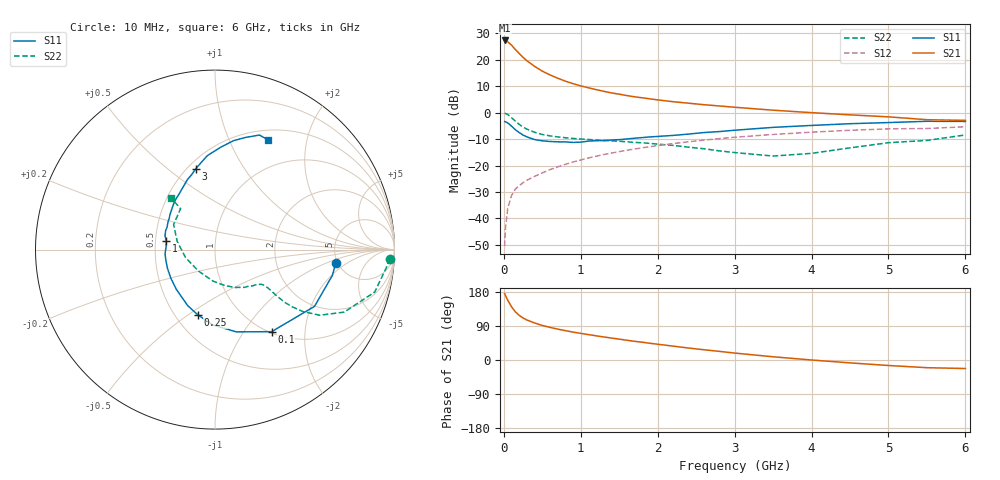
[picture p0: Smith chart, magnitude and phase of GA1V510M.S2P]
! Infineon Technologies  Discrete & RF Semiconductors
! BF775
! Si NPN RF Bipolar Junction Transistor in SOT23
! VCE = 1.5 V  IC = 10 mA
! Common Emitter S-Parameters:  May  1996
# GHz  S  MA  R  50
!  f  S11  S21  S12  S22
! GHz  MAG  ANG  MAG  ANG  MAG  ANG  MAG  ANG
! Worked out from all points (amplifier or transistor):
!   36 points, 10 MHz to 6 GHz, reference 50 ohm
!   highest |S21| = 27.2 dB at 10 MHz (marker M1)
!   |S21| within 3 dB of that: start of sweep to 137.2 MHz
!   unconditionally stable (mu >= 1): 496 MHz to 4.195 GHz; 5.231 GHz to end of sweep
!   at 250 MHz: K = 0.72, MSG = 23.7 dB, |S12| = -26.5 dB
!   at 1.4 GHz: K = 1.14, MAG = 9.1 dB, |S12| = -15.3 dB
!   at 6 GHz: K = 1.00, MAG = 0.9 dB, |S12| = -5.4 dB
!   S11 on the Smith chart (normalised r, x): 10 MHz: 4.79, -1.33; 100 MHz: 1.02, -1.35; 250 MHz: 0.64, -0.54; 1 GHz: 0.57, +0.06; 3 GHz: 0.55, +0.63; 6 GHz: 0.62, +1.41
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0.01  0.6762 -6.4  22.98 175.5  0.003 87.1  0.9741 -3.0
0.02  0.6699 -12.3  22.75 170.7  0.0063 86.0  0.959 -6.2
0.05  0.6383 -29.7  21.82 158.1  0.0154 76.9  0.9205 -14.9
0.1  0.5556 -55.4  18.73 140.4  0.0271 67.3  0.8001 -25.8
0.15  0.4734 -75.5  15.5 127.0  0.0359 61.8  0.688 -32.1
0.2  0.4188 -92.0  13.02 117.7  0.0418 60.1  0.5977 -35.2
0.25  0.3757 -104.8  11.02 110.8  0.0473 59.1  0.5323 -36.6
0.3  0.3475 -115.9  9.505 105.5  0.0528 59.4  0.4869 -37.1
0.4  0.3088 -134.3  7.457 97.7  0.0624 60.6  0.4237 -36.8
0.5  0.2927 -147.5  6.053 91.2  0.0725 61.5  0.3851 -36.2
0.6  0.2844 -158.8  5.132 86.1  0.0836 62.1  0.3633 -35.9
0.7  0.2802 -167.7  4.454 81.5  0.0943 62.6  0.3473 -35.9
0.8  0.2792 -175.4  3.915 77.5  0.1052 62.5  0.3346 -36.2
1  0.2764 169.8  3.19 70.3  0.1274 62.1  0.3171 -37.5
1.1  0.289 164.5  2.933 67.0  0.1388 61.7  0.3103 -38.9
1.6  0.3172 142.3  2.09 52.1  0.1943 57.4  0.28 -47.0
2.2  0.3701 122.5  1.603 36.6  0.2597 50.7  0.2402 -61.5
3  0.464 103.3  1.259 18.3  0.3415 40.3  0.1757 -93.7
3.5  0.525 94.7  1.108 8.5  0.386 33.3  0.151 -127.6
4.5  0.616 80.3  0.905 -7.6  0.4627 19.7  0.2154 167.9
5.5  0.6845 68.8  0.733 -20.3  0.5001 5.6  0.2976 130.1
6  0.6793 64.0  0.712 -22.5  0.5393 1.5  0.378 130.3
